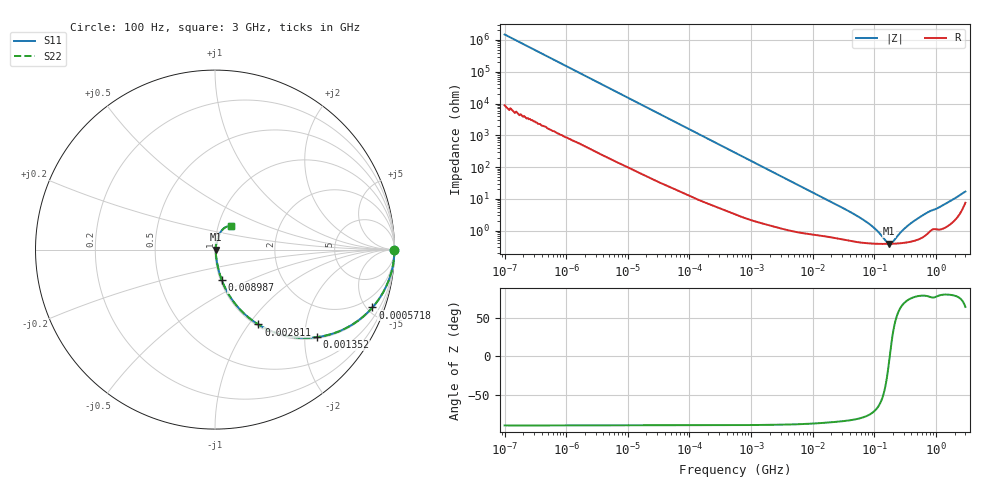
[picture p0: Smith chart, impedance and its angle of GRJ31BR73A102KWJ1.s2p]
!Murata Part Number: GRJ31BR73A102KWJ1
!These Parameters are Measured in Series Mode Connection
!Data Generated on Jun 19, 2026
!  o--ll--o
!Port1  Port2
!  o------o
!Operation Temp=25[degC], DC Bias Voltage=0[V]
!Freq. Start=100[Hz] Stop=3[GHz] 401[Steps]
# Hz S RI R 50
!Freq.(Hz) S11(Real) S11(Imag) S21(Real) S21(Imag) S12(Real) S12(Imag) S22(Real) S22(Imag)
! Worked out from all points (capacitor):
!   401 points, 100 Hz to 3 GHz, reference 50 ohm
!   read as one part in series: C = 1.07 nF near 109 Hz
!   lowest |Z| = 385 mohm at 175.1 MHz (marker M1)
!   series resonance near 177.9 MHz, so ESL is about 750 pH
!   S11 on the Smith chart (normalised r, x): 100 Hz: open; 571.8 kHz: 1.06, -5.42; 1.352 MHz: 1.04, -2.30; 2.811 MHz: 1.02, -1.11; 8.987 MHz: 1.02, -0.35; 3 GHz: 1.15, +0.30
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100  1 -6.7e-05  4e-07 6.7e-05  4e-07 6.7e-05  1 -6.7e-05
161  1 -0.000107  6e-07 0.000107  6e-07 0.000107  1 -0.000107
1788  1 -0.00119  8.5e-06 0.00119  8.5e-06 0.00119  1 -0.00119
31977  0.9994 -0.0209  0.000586 0.0209  0.000586 0.0209  0.9994 -0.0209
164120  0.9878 -0.1054  0.0122 0.1054  0.0122 0.1054  0.9878 -0.1054
547723  0.8859 -0.3122  0.1141 0.3122  0.1141 0.3122  0.8859 -0.3122
571812  0.8771 -0.3225  0.1229 0.3225  0.1229 0.3225  0.8771 -0.3225
879390  0.7541 -0.4241  0.2459 0.4241  0.2459 0.4241  0.7541 -0.4241
1352413  0.5687 -0.4875  0.4313 0.4875  0.4313 0.4875  0.5687 -0.4875
2811170  0.2415 -0.4172  0.7585 0.4172  0.7585 0.4172  0.2415 -0.4172
4711951  0.1069 -0.295  0.8931 0.295  0.8931 0.295  0.1069 -0.295
8986547  0.037 -0.1679  0.963 0.1679  0.963 0.1679  0.037 -0.1679
9794414  0.0323 -0.155  0.9677 0.155  0.9677 0.155  0.0323 -0.155
6.794454e7  0.00452 -0.0207  0.9955 0.0207  0.9955 0.0207  0.00452 -0.0207
1.000898e8  0.004 -0.0113  0.996 0.0113  0.996 0.0113  0.004 -0.0113
1.539281e8  0.00381 -0.0027  0.9962 0.0027  0.9962 0.0027  0.00381 -0.0027
1.751444e8  0.00382 -0.000286  0.9962 0.000286  0.9962 0.000286  0.00382 -0.000286
1.99285e8  0.00386 0.00213  0.9961 -0.00213  0.9961 -0.00213  0.00386 0.00213
3.064804e8  0.00424 0.0107  0.9958 -0.0107  0.9958 -0.0107  0.00424 0.0107
4.920662e8  0.00557 0.0225  0.9944 -0.0225  0.9944 -0.0225  0.00557 0.0225
1.789813e9  0.0242 0.0851  0.9758 -0.0851  0.9758 -0.0851  0.0242 0.0851
3e9  0.0881 0.129  0.9119 -0.129  0.9119 -0.129  0.0881 0.129
